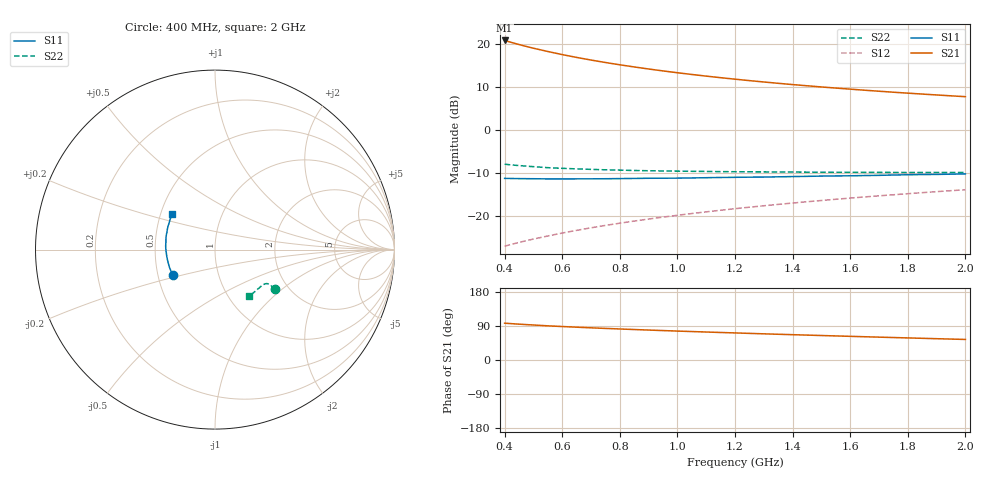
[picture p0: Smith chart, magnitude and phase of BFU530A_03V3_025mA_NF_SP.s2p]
! Filename:  P:\Prog\Test\Noise\ATS_data\Testdata_Net\06 Compressed Noise after Statistics\BFU530A_APG2013_33_A05_03p3V_025mA_NF_CM01_D.sf
! Date/Time: Tue 16/Apr/2013 15:11:06
! BFU530A_APG2013_33_A05_03p3V_1to25mA_NF_CM01_Bias8_R.sf
! Noise Parameter Data File
! BFU530A_APG2013_33_A05_03p3V_1to25mA_NF_CM01
! Date/time: Fri Apr 12 14:21:19 2013
! VAR V_out= 3.300000
! VAR I_out= 24.995000
! VAR V_in= 0.854600
! VAR I_in= 0.285650
! Device data file deembeded for feedlines and parallel
! Original file: \06 Compressed Noise after Statistics\BFU530A_APG2013_33_A05_03p3V_025mA_NF_CM01_R.sf
! Feed-files: PR017V01_150413_Feed1.s2p, PR017V01_150413_Feed2.s2p
! Parallel-file: PR017V01_150413_Par.s2p
# MHz S MA R 50
!  Freq-MHz  S11-mag  S11-arg  S21-mag  S21-arg  S12-mag  S12-arg  S22-mag  S22-arg
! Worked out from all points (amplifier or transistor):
!   37 points, 400 MHz to 2 GHz, reference 50 ohm
!   highest |S21| = 20.8 dB at 400 MHz (marker M1)
!   |S21| within 3 dB of that: start of sweep to 580.6 MHz
!   unconditionally stable (mu >= 1): 707.1 MHz to 1.731 GHz
!   at 500 MHz: K = 0.96, MSG = 22.1 dB, |S12| = -25.3 dB
!   at 1.1 GHz: K = 1.02, MAG = 15.0 dB, |S12| = -19.0 dB
!   at 2 GHz: K = 0.99, MSG = 10.8 dB, |S12| = -13.9 dB
!   lowest NFmin = 1.13 dB at 420 MHz
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400  0.2744 -149.6  10.93 97.2  0.04492 72.3  0.4009 -33.4
420  0.274 -151.8  10.45 96.1  0.04681 72.6  0.3945 -33.3
440  0.2732 -153.9  10.01 95.1  0.04871 72.8  0.3891 -33.1
480  0.2724 -157.7  9.227 93.2  0.05243 73.2  0.3794 -32.9
500  0.2721 -159.5  8.881 92.3  0.05431 73.4  0.3755 -32.8
550  0.2708 -163.7  8.134 90.2  0.05897 73.8  0.3656 -32.6
600  0.2709 -167.2  7.491 88.3  0.06378 74.0  0.3592 -32.6
650  0.2711 -170.5  6.946 86.6  0.06853 74.2  0.3538 -32.8
700  0.2713 -173.4  6.476 84.9  0.07335 74.4  0.3493 -33.0
750  0.272 -176.4  6.063 83.4  0.0782 74.5  0.3453 -33.2
800  0.2731 -178.9  5.704 81.9  0.083 74.5  0.3424 -33.7
850  0.2743 178.5  5.385 80.4  0.08783 74.4  0.339 -34.1
900  0.2755 176.1  5.099 79.0  0.09271 74.4  0.3366 -34.6
950  0.2759 173.9  4.844 77.7  0.09756 74.3  0.335 -35.2
1050  0.2779 169.8  4.404 75.1  0.1074 74.1  0.3317 -36.4
1150  0.2813 165.8  4.042 72.6  0.1173 73.7  0.3288 -37.8
1200  0.2824 164.1  3.885 71.4  0.1222 73.5  0.3281 -38.6
1350  0.2863 158.9  3.479 67.9  0.1371 72.8  0.3261 -41.1
1500  0.292 154.0  3.156 64.6  0.1521 72.0  0.3236 -43.7
1650  0.2962 149.6  2.893 61.4  0.1673 71.0  0.3228 -46.6
1750  0.3004 146.7  2.742 59.3  0.1773 70.3  0.3219 -48.6
2000  0.3096 140.1  2.434 54.3  0.2028 68.5  0.3215 -53.9
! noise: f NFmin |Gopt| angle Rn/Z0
400  1.179  0.325  -167.7  0.078
460  1.146  0.3288  -165.1  0.0783
600  1.251  0.3261  -155.4  0.0911
800  1.237  0.3674  -156  0.077
1000  1.222  0.3817  -149.6  0.0859
1200  1.296  0.3997  -143.9  0.092
1400  1.321  0.413  -140.1  0.1016
1600  1.342  0.4401  -133.6  0.115
1800  1.314  0.4695  -127.8  0.132
2000  1.4  0.4537  -122.8  0.1542
